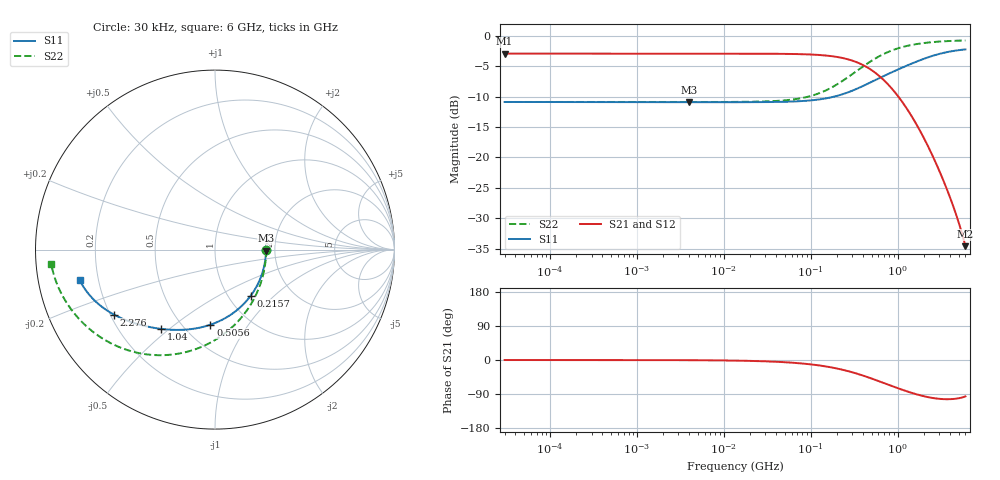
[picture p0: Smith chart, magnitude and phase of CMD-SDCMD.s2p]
!EMIF06-MSD04F3
!Simulation
!24/03/11  09:04
!Start Freq. :30.000kHz; Stop Freq. : 6.000GHz
!Number of points : 1592; Sweep : LOGARITHMIC
!C1-C4 (CMD-SDCMD)
!Freq ReS11 ImS11 ReS21 ImS21 ReS12 ImS12 ReS22 ImS22
# Hz  S  RI  R  50
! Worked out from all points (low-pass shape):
!   1592 points, 30 kHz to 6 GHz, reference 50 ohm
!   highest |S21| = -2.92 dB at 30 kHz (marker M1); lowest = -34.6 dB at 6 GHz (marker M2)
!   |S21| within 3 dB of the highest: start of sweep to 533.3 MHz
!   lowest |S11| = -10.9 dB at 3.955 MHz (marker M3), VSWR 1.79, Z = 89.7 - j1.05 ohm
!   |S11| at or under -10 dB: start of sweep to 186.1 MHz
!   |S22| runs from -10.9 to -0.8 dB; largest |S21 - S12| = 2e-15
!   S11 on the Smith chart (normalised r, x): 30 kHz: 1.80, -0.00; 215.7 MHz: 1.26, -0.73; 505.6 MHz: 0.67, -0.68; 1.04 GHz: 0.38, -0.47; 2.276 GHz: 0.22, -0.28; 6 GHz: 0.13, -0.11
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30000  0.2855 -0.000524  0.7142 -0.000312  0.7142 -0.000312  0.2857 -0.000211
231093.6  0.2844 -0.000816  0.7135 -0.000615  0.7135 -0.000615  0.2853 -0.000631
1766531  0.2841 -0.00251  0.7134 -0.00264  0.7134 -0.00264  0.2852 -0.00367
3954770  0.2841 -0.00539  0.7133 -0.00577  0.7133 -0.00577  0.2852 -0.00815
1.350376e7  0.2837 -0.0182  0.7129 -0.0196  0.7129 -0.0196  0.2846 -0.0277
4.336319e7  0.2801 -0.058  0.7084 -0.0624  0.7084 -0.0624  0.2785 -0.0885
6.820056e7  0.2744 -0.0905  0.7012 -0.0973  0.7012 -0.0973  0.2687 -0.1381
1.032257e8  0.2623 -0.1349  0.6861 -0.1445  0.6861 -0.1445  0.2482 -0.2053
1.538584e8  0.2375 -0.1946  0.655 -0.2069  0.655 -0.2069  0.206 -0.2946
2.156691e8  0.1979 -0.2583  0.6059 -0.2711  0.6059 -0.2711  0.1391 -0.3877
3.239325e8  0.115 -0.343  0.5044 -0.3486  0.5044 -0.3486  0.000475 -0.5036
4.10949e8  0.0455 -0.388  0.4215 -0.3812  0.4215 -0.3812  -0.1138 -0.5567
5.055777e8  -0.026 -0.4187  0.3389 -0.3937  0.3389 -0.3937  -0.2286 -0.5835
6.267888e8  -0.107 -0.4391  0.2502 -0.387  0.2502 -0.387  -0.354 -0.5864
7.890804e8  -0.1961 -0.4473  0.1616 -0.3576  0.1616 -0.3576  -0.4832 -0.5614
1.040211e9  -0.3001 -0.4418  0.0761 -0.2996  0.0761 -0.2996  -0.6166 -0.5015
1.503562e9  -0.4297 -0.4155  0.00752 -0.208  0.00752 -0.208  -0.7462 -0.3982
2.275733e9  -0.5618 -0.3627  -0.0175 -0.1186  -0.0175 -0.1186  -0.8348 -0.2829
3e9  -0.6366 -0.3137  -0.0168 -0.076  -0.0168 -0.076  -0.8704 -0.215
3.894526e9  -0.6929 -0.2604  -0.0114 -0.0478  -0.0114 -0.0478  -0.8924 -0.1583
4.75468e9  -0.726 -0.2182  -0.00676 -0.0322  -0.00676 -0.0322  -0.9037 -0.1194
6e9  -0.7545 -0.1699  -0.00196 -0.0185  -0.00196 -0.0185  -0.9126 -0.078
